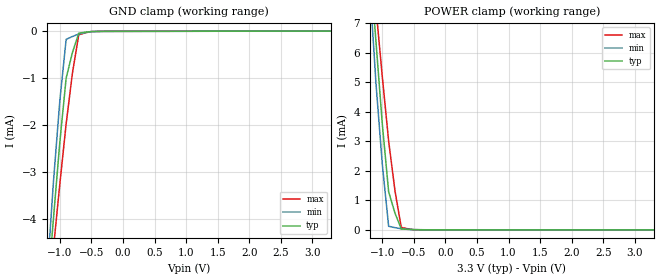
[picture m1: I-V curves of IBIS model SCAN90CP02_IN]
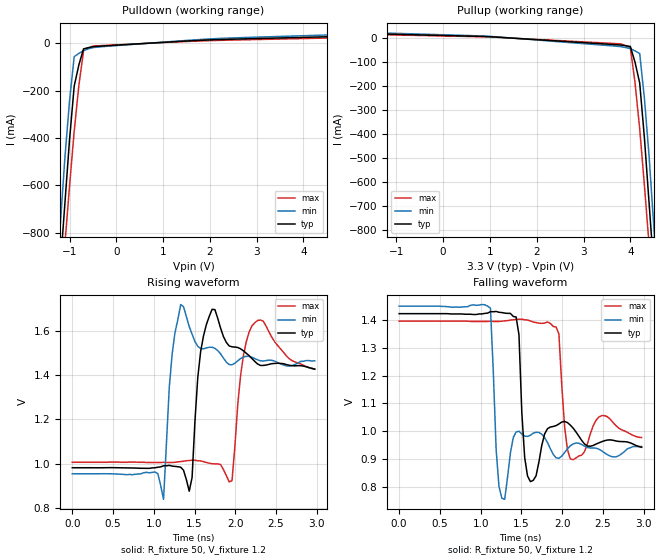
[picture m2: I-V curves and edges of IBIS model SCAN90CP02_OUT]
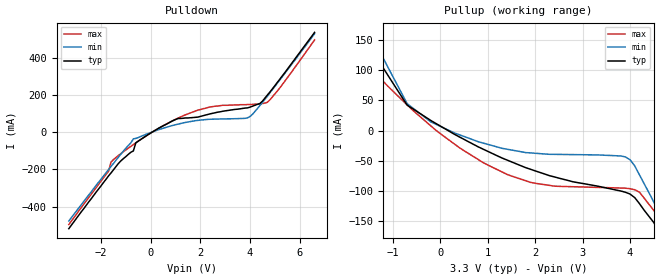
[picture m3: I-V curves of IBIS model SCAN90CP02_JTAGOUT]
|   National Semiconductor Corporation
|   IBIS Model
|   of
|   SCAN90CP02
|   1.5Gbps 2x2 LVDS Crosspoint Switch
|   with Pre-emphasis and IEEE1149.6
|   28 pin LLP package
[IBIS Ver]   3.2
[Comment Char]   |_char
[File name]   scan90cp02_pem.ibs
[File Rev]   1.0
[Date]   10/25/03
[Source]
SpectreS simulation, Bench data
IEEE1149.1 cells created from SCAN928028
[Notes]
Created by Ivan Duzevik
[Disclaimer]
(C) Copyright National Semiconductor Corporation 2002
   All rights reserved
   National Semiconductor Corporation hereby grants
the user of this IBIS model a non-exclusive, nontransferable
license to use this IBIS model under the following terms.
Before using this IBIS model, the user should read this
license.  If the user does not accept these terms,  the
IBIS model should be returned to National within 30 days.
   The user is granted this license only to use the
IBIS model and is not granted rights to sell, load, rent,
lease or license the IBIS model in whole or in part, or in
modified form to anyone other than user. User may modify
the IBIS model to suit its specific applications but rights
to derivative works and such modifications shall belong to
National.
   This IBIS model is provided on an "AS IS" basis and
National makes absolutely no warranty with respect to the
information contained herein.NATIONAL DISCLAIMS AND CUSTOMER
WAIVES ALL WARRANTIES, EXPRESS OR IMPLIED, INCLUDING
WARRANTIES OF MERCHANTABILITY OR FITNESS FOR A PARTICULAR
PURPOSE. The entire risk as to quality and performance is
with the Customer. ACCORDINGLY, IN NO EVENT SHALL THE
COMPANY BE LIABLE FOR ANY DAMAGES, WHETHER IN CONTRACT OR
TORT,INCLUDING ANY LOST PROFITS OR OTHER INCIDENTAL,
CONSEQUENTIAL, EXEMPLARY, OR PUNITIVE DAMAGES ARISING OUT
OF THE USE OR APPLICATION OF THE IBIS model provided in
this package.Further, National reserves the right to make
changes without notice to any product herein to improve
reliability, function, or design. National does not convey
any license under patent rights or any other intellectual
property rights, including those of third parties.
   National is not obligated to provide maintenance or support
for the licensed IBIS model.
Contact National at ATTN:ENHANCED SOLUTIONS/IBIS MODELS.
5 Foden Road, M/S 01-50, South Porltand, ME 04106
(207) 541-8467
[Copyright]
(c) Copyright 2002 National Semiconductor Corp.
[Component]   SCAN90CP02
Si_location Pin
Timing_location Pin
[Manufacturer]   National Semiconductor Corp.
[Package]
|   TYP   MIN   MAX
R_pkg   100.0m   100.0m   100.0m
L_pkg   1nH   1nH   1nH
C_pkg   0.2pF   0.2pF   0.2pF
[Pin]   signal_name   model_name   R_pin   L_pin   C_pin
1   PEM11   SCAN90CP02_SEL
2   PEM10   SCAN90CP02_SEL
3   PEM01   SCAN90CP02_SEL
4   PEM00   SCAN90CP02_SEL
5   SEL1   SCAN90CP02_SEL
6   SEL0   SCAN90CP02_SEL
7   EN0b   SCAN90CP02_SEL
8   NC   NC
9   IN0+   SCAN90CP02_IN
10   IN0-   SCAN90CP02_IN
11   VDDA   POWER
12   IN1+   SCAN90CP02_IN
13   IN1-   SCAN90CP02_IN
14   VDD2   POWER
15   EN1b   SCAN90CP02_SEL
16   VDD1   POWER
17   TCK   SCAN90CP02_SEL
18   TMS   SCAN90CP02_SEL
19   TDI   SCAN90CP02_SEL
20   TDO   SCAN90CP02_JTAGOUT
21   TRSTb   SCAN90CP02_SEL
22   VDD2   POWER
23   OUT1-   SCAN90CP02_OUT
24   OUT1+   SCAN90CP02_OUT
25   VDDA   POWER
26   OUT0-   SCAN90CP02_OUT
27   OUT0+   SCAN90CP02_OUT
28   NC   NC
[Diff Pin] inv_pin   vdiff   tdelay_typ   tdelay_min   tdelay_max
| The '+' pin is Diff_pin and the '-' pin is the inv_pin
| Receiver Vth = +/-100mV
9   10   0.05   0   0   0
12   13   0.05   0   0   0
| Models and submodels in the file (4): SCAN90CP02_IN (Input), SCAN90CP02_OUT (Output), SCAN90CP02_JTAGOUT (Output), SCAN90CP02_SEL (Input)
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[Model]   SCAN90CP02_IN
Model_type Input
Vinh=0.05
Vinl=-0.05
C_comp   5pF   5pF   5pF
[Temperature Range] 25   -40   85
[Voltage Range]   3.3   3.3   3.3
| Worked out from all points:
|   GND clamp passes 1 mA (typ) near -0.90 V on its own axis
|   POWER clamp passes 1 mA (typ) near -0.86 V on its own axis
[GND Clamp]
|V(groundclamp)   I(typ)   I(max)   I(min)
-3.3V     -39.4mA    -48.4mA    -34.1mA
-1.2V     -5.59mA    -5.16mA    -5.94mA
-1.1V     -3.97mA    -3.18mA    -4.6mA
-1V       -2.36mA    -1.48mA    -3.25mA
-900mV    -999uA     -174uA     -1.97mA
-800mV    -452uA     -113uA     -888uA
-700mV    -42uA      -60.2uA    -77.3uA
-500mV    -8.18uA    -10.7uA    -6.08uA
3.3V      1.65uA     2.08uA     1.37uA
[POWER Clamp]
|Vtable   I(typ)   I(max)   I(min)
-3.3V     67.6mA     82.8mA     58.5mA
-1.2V     9.15mA     8.31mA     9.82mA
-1.1V     6.36mA     4.94mA     7.5mA
-1V       3.58mA     2.21mA     5.18mA
-900mV    1.29mA     121uA      3.01mA
-800mV    569uA      75.2uA     1.33mA
-700mV    31.3uA     36.8uA     82.2uA
-500mV    6.39uA     7.01uA     5.42uA
3.3V      -3.3uA     -4.15uA    -2.73uA
[Model]   SCAN90CP02_OUT
Model_type Output
Polarity Inverting
Vref=1.20
Rref=50   | 100 Ohms Across Outputs OUTP and OUTM
Cref=1p
C_comp   8pF   8pF   8pF
[Temperature Range] 25   -40   85
[Voltage Range]   3.3   3.3   3.3
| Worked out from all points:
|   slope of the pulldown table from 0 to 0.495 V, typ, clamps not added: 83.8 ohm
|   slope of the pullup table from 0 to 0.495 V, typ, clamps not added: 205 ohm
|   falling waveform, R_fixture 50, V_fixture 1.2: 20-80 % time 38.9ps typ, 41.6ps min, 52.3ps max; typ from 1.42 V to 0.942 V
|   rising waveform, R_fixture 50, V_fixture 1.2: 20-80 % time 42.5ps typ, 44ps min, 53ps max; typ from 0.981 V to 1.43 V
[Pulldown]
|V(pulldown)   I(typ)   I(max)   I(min)
-3.3V     -6.656A    -7.152A    -6.291A
-1.3V     -1.224A    -1.081A    -1.347A
-1.2V     -952.2mA   -777.6mA   -1.1A
-1.1V     -680.3mA   -487.1mA   -852.4mA
-1V       -408.7mA   -244mA     -605.4mA
-900mV    -180.7mA   -55.84mA   -371.2mA
-800mV    -90.66mA   -42.04mA   -177.5mA
-700mV    -22.76mA   -30.04mA   -31.19mA
-500mV    -13.84mA   -17.61mA   -11.18mA
1.2V      6.881mA    8.468mA    5.664mA
5.6V      34.78mA    43.71mA    28.24mA
6.6V      44.32mA    56.85mA    35.62mA
[Pullup]
|V(pullup)   I(typ)   I(max)   I(min)
-3.3V     27.3mA     33.4mA     22.6mA
1.1V      5.23mA     6.35mA     4.67mA
3.8V      -28.34mA   -34.94mA   -23.46mA
4V        -34.39mA   -43.15mA   -40.11mA
4.1V      -99.67mA   -52.59mA   -185mA
4.2V      -186.7mA   -63.76mA   -377.4mA
4.3V      -413.5mA   -249.4mA   -611.5mA
4.4V      -684.5mA   -490.1mA   -858.8mA
4.5V      -956.3mA   -779.4mA   -1.107A
4.6V      -1.228A    -1.082A    -1.354A
6.6V      -6.675A    -7.166A    -6.313A
[Falling Waveform]
R_fixture=50
V_fixture=1.2
V_fixture_min=1.2
V_fixture_max=1.2
0s        1.423V     1.45V      1.396V
1.12ns    1.43V      1.443V     1.396V
1.19ns    1.431V     933.8mV    1.395V
1.26ns    1.427V     758.8mV    1.396V
1.435ns   1.411V     997.2mV    1.402V
1.54ns    905.4mV    982.4mV    1.401V
1.61ns    818.6mV    985.3mV    1.397V
1.96ns    1.026V     902.4mV    1.35V
2.1ns     1.022V     947.5mV    900.3mV
2.975ns   942mV      944.9mV    977.3mV
[Rising Waveform]
R_fixture=50
V_fixture=1.2
V_fixture_min=1.2
V_fixture_max=1.2
0s        981.4mV    954.2mV    1.006V
1.12ns    990.2mV    838.8mV    1.006V
1.225ns   988.9mV    1.494V     1.005V
1.33ns    983.9mV    1.718V     1.009V
1.47ns    937.6mV    1.584V     1.015V
1.575ns   1.506V     1.519V     1.012V
1.715ns   1.696V     1.525V     999.6mV
1.96ns    1.527V     1.446V     923.4mV
2.24ns    1.461V     1.474V     1.636V
2.975ns   1.426V     1.464V     1.427V
[Ramp]
|   typ   max   min
dV/dt_r   312mV/0.043ns   313mV/0.046ns   306mV/0.063ns
dV/dt_f   306mv/0.037ns   313mv/0.027ns   312mv/0.074ns
R_load=50
|[End   SCAN90CP02_OUT
[Model]   SCAN90CP02_JTAGOUT
Model_type Output
Polarity Non-Inverting
Vref=0.0
Vmeas=1.65
Rref=500
Cref=50p
C_comp   5pF   5pF   5pF
[Temperature Range] 25   -40   85
[Voltage Range]   3.3   3.6   3.0
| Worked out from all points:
|   slope of the pulldown table from 0 to 0.495 V, typ, clamps not added: 12.9 ohm
|   slope of the pullup table from 0 to 0.495 V, typ, clamps not added: 22.7 ohm
[Pullup]
|Vtable   I(typ)   I(max)   I(min)
-3.3V     539mA      529mA      495mA
-1.7V     187mA      200mA      202mA
-1.5V     153mA      168mA      170mA
-1.4V     137mA      151mA      159mA
-1.3V     120mA      135mA      89.1mA
-700mV    42mA       44.5mA     42.5mA
300mV     -6.33mA    -4.05mA    -22.5mA
1.4V      -48.6mA    -30.8mA    -72.3mA
3.9V      -102mA     -43.6mA    -95.3mA
4.2V      -121mA     -73.5mA    -102mA
4.8V      -200mA     -167mA     -172mA
6.6V      -516mA     -476mA     -495mA
[Pulldown]
|V(pulldown)   I(typ)   I(max)   I(min)
-3.3V     -518mA     -477mA     -496mA
-1.7V     -235mA     -201mA     -210mA
-1.6V     -219mA     -184mA     -161mA
-1.2V     -154mA     -118mA     -115mA
-700mV    -101mA     -36.2mA    -66.9mA
-600mV    -57.4mA    -33.7mA    -57.4mA
1.1V      72.9mA     42.8mA     74.9mA
2.4V      98.3mA     69mA       135mA
4V        134mA      83.9mA     148mA
4.4V      154mA      143mA      151mA
4.8V      215mA      211mA      173mA
6.6V      535mA      528mA      495mA
[Ramp]
|   typ   max   min
dV/dt_r   1.26V/.185ns   0.96V/.200ns   1.5V/.060ns
dV/dt_f   1.45V/.240ns   1.15V/.260ns   1.64V/.12ns
R_load=50
|[End   SCAN90CP02_JTAGOUT
